(* Logix 5000 DataType export RSG3E_Seneca_OutData; software revision 35.00 *)

TYPE RSG3E_Seneca_OutData :   // User Define Data Out Type for Seneca R-SG3-E Device
STRUCT
   DOUT1 : BOOL;   // Digital Output1
   DOUT2 : BOOL;   // Digital Output2
   CMD : INT;   // Command Register
   CMD_AUX : UDINT;   // Command Auxiliar
   PARAM_FORCE_CFG : INT;
   PARAM_DELTA_T : INT;
   PARAM_FM : SINT;
   PARAM_MT : SINT;
   PARAM_MU : SINT;
   PARAM_RESOLUTION : SINT;
   PARAM_NOISE_FILTER : SINT;
   PARAM_FILTER_LEVEL : SINT;
   PARAM_AUTOMATIC_TARE : SINT;
   PARAM_ADC_SPEED : SINT;
   PARAM_CELL : REAL;
   PARAM_FS : REAL;
   PARAM_STD_W : REAL;
   PARAM_NOISE_VAR : REAL;
   PARAM_FILTER_RESP_VEL : REAL;
   PARAM_MAN_RESOLUTION : REAL;
   PARAM_SAMPLE_PIECE_W : REAL;
   PARAM_TARE_W : UDINT;
   PARAM_DELTA_W : REAL;
   PARAM_IO_MODE1 : SINT;
   PARAM_IO_FUNC1 : SINT;
   PARAM_DOUT_MODE1 : SINT;
   PARAM_DOUT_CONF1 : SINT;
   PARAM_THRESHOLD1 : REAL;
   PARAM_HYSTERESIS1 : REAL;
   PARAM_IO_MODE2 : SINT;
   PARAM_IO_FUNC2 : SINT;
   PARAM_DOUT_MODE2 : SINT;
   PARAM_DOUT_CONF2 : SINT;
   PARAM_THRESHOLD2 : REAL;
   PARAM_HYSTERESIS2 : REAL;
END_STRUCT
END_TYPE
